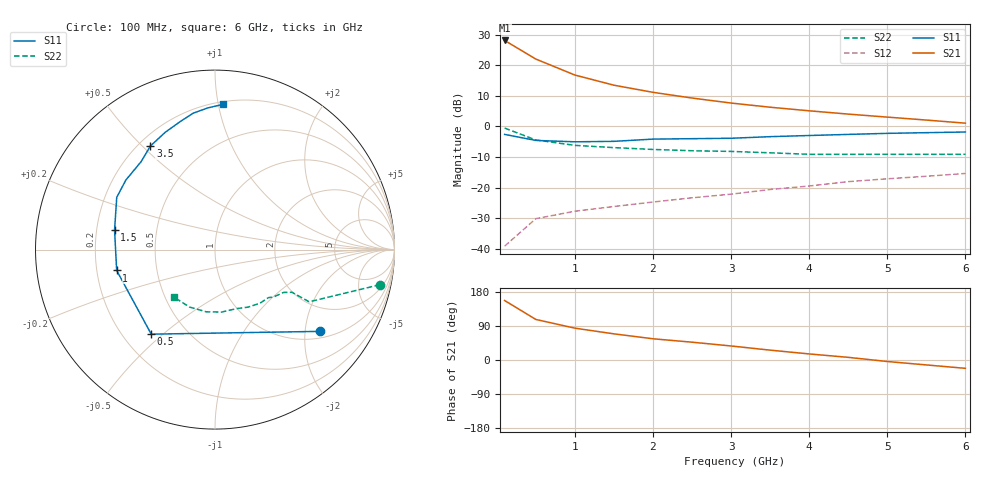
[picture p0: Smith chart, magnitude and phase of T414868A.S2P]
!AT-41486
!S AND NOISE PARAMETERS at Vce=8V  Ic=10mA.  LAST UPDATED 07-21-92
# ghz s ma r 50
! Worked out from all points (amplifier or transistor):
!   13 points, 100 MHz to 6 GHz, reference 50 ohm
!   highest |S21| = 28.1 dB at 100 MHz (marker M1)
!   |S21| within 3 dB of that: start of sweep to 297.1 MHz
!   unconditionally stable (mu >= 1): 1.415 GHz to 4.015 GHz
!   at 1 GHz: K = 0.83, MSG = 22.3 dB, |S12| = -27.7 dB
!   at 3 GHz: K = 1.18, MAG = 12.3 dB, |S12| = -22.2 dB
!   at 6 GHz: K = 0.72, MSG = 8.2 dB, |S12| = -15.4 dB
!   lowest NFmin = 1.30 dB at 100 MHz
!   S11 on the Smith chart (normalised r, x): 100 MHz: 1.19, -2.39; 500 MHz: 0.32, -0.46; 1 GHz: 0.28, -0.10; 1.5 GHz: 0.28, +0.09; 3.5 GHz: 0.25, +0.53; 6 GHz: 0.22, +1.03
0.1  0.74 -38.0  25.46 157.0  0.011 68.0  0.94 -12.0
0.5  0.59 -127.0  12.63 107.0  0.031 47.0  0.6 -29.0
1  0.56 -168.0  6.92 84.0  0.041 46.0  0.49 -29.0
1.5  0.57 169.0  4.72 69.0  0.049 49.0  0.45 -32.0
2  0.62 152.0  3.61 56.0  0.058 43.0  0.42 -39.0
2.5  0.63 142.0  2.91 47.0  0.068 52.0  0.4 -42.0
3  0.64 130.0  2.41 37.0  0.078 52.0  0.39 -50.0
3.5  0.68 122.0  2.06 26.0  0.093 51.0  0.37 -60.0
4  0.71 113.0  1.8 16.0  0.106 48.0  0.35 -70.0
4.5  0.74 105.0  1.59 7.0  0.125 48.0  0.35 -84.0
5  0.77 99.0  1.42 -4.0  0.139 43.0  0.35 -98.0
5.5  0.79 93.0  1.27 -13.0  0.153 38.0  0.35 -114.0
6  0.81 87.0  1.13 -22.0  0.17 34.0  0.35 -131.0
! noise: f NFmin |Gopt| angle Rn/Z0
0.1  1.3  0.12  3  0.17
0.5  1.3  0.1  16  0.17
1  1.4  0.04  43  0.16
2  1.7  0.12  -145  0.16
4  3  0.44  -99  0.4
